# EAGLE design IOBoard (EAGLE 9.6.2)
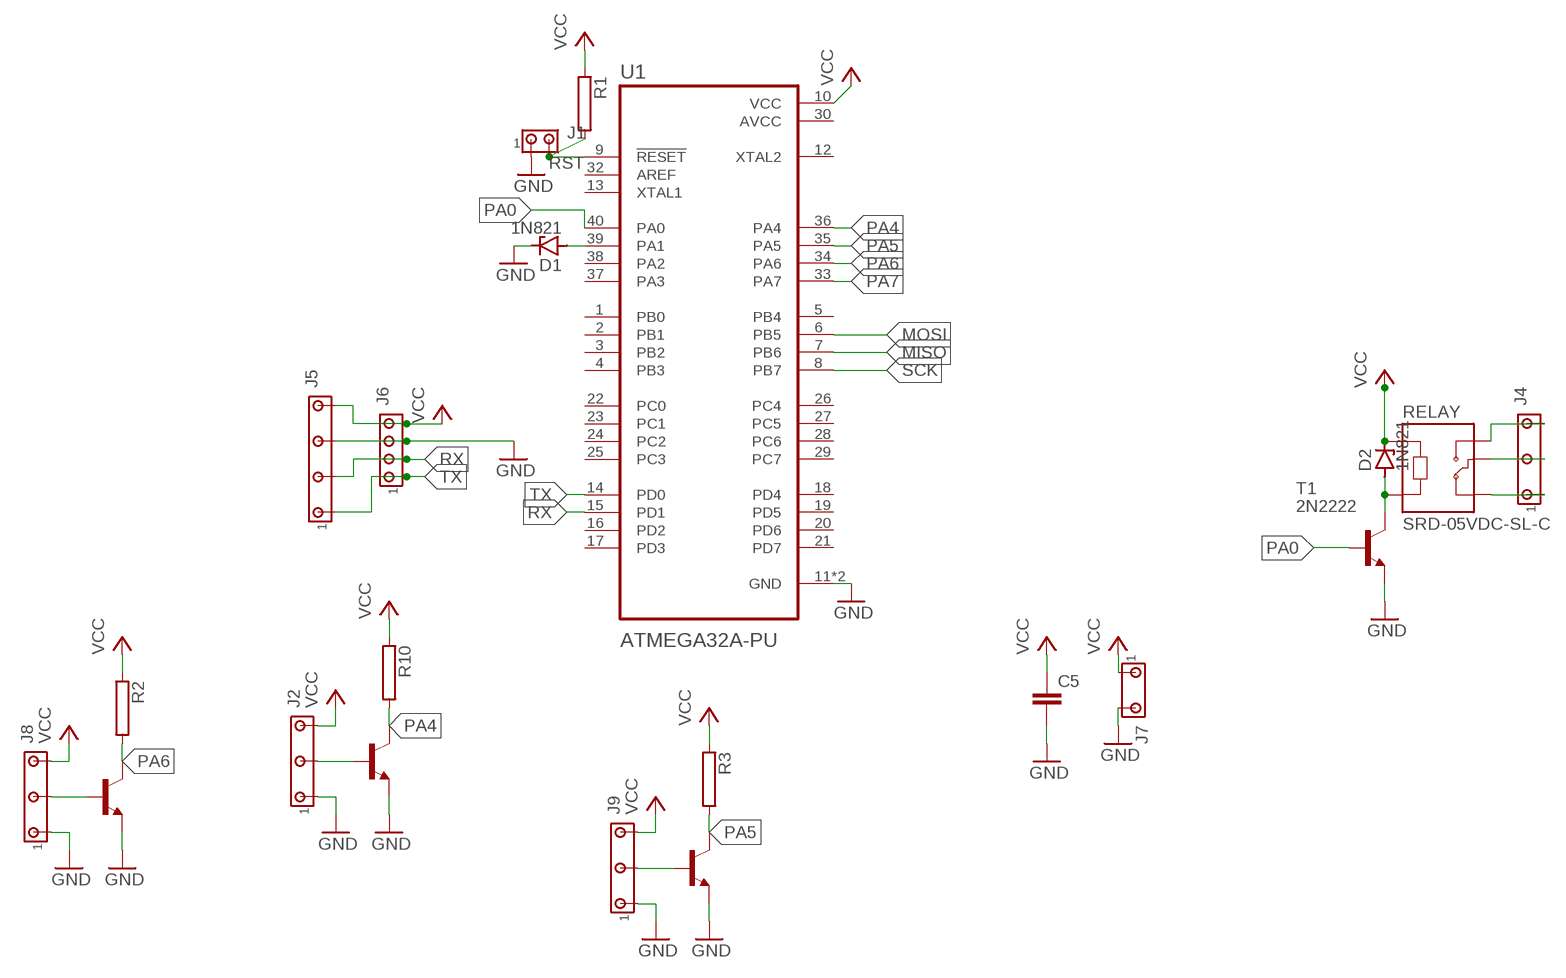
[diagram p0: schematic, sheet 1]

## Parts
C5  C-EU025-024X044  [C025-024X044]
D1  1N821  [DO35Z10]
D2  1N821  [DO35Z10]
J1  MTA02-100  [10X02MTA]
J2  MTA05-156_MYVSPACE1  [10X05MTA_MYV]
J4  MTA05-156_MYVSPACE1  [10X05MTA_MYV]
J5  MTA07-100_MYV  [10X07MTA_MYV]
J6  MTA04-100  [10X04MTA]
J7  MTA03-100_MYV  [10X03MTA_MYV]
J8  MTA05-156_MYVSPACE1  [10X05MTA_MYV]
J9  MTA05-156_MYVSPACE1  [10X05MTA_MYV]
R1  RHPS58  [HPS58]
R2  RHPS58  [HPS58]
R3  RHPS58  [HPS58]
R10  RHPS58  [HPS58]
RELAY  SRD-05VDC-SL-C  [RELAY_SRD-05VDC-SL-C]
T1  2N2222  [TO18]
T2  2N2222  [TO18]
T5  2N2222  [TO18]
T6  2N2222  [TO18]
U1  ATMEGA32A-PU  [DIP1540W47P254L5320H635Q40B]

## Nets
GND: C5.2 D1.C J1.1 J2.1 J5.5 J6.3 J7.3 J8.1 J9.1 T1.1(E) T2.1(E) T5.1(E) T6.1(E) U1.11(GND) U1.31(GND)
MISO: U1.7(PB6)
MOSI: U1.6(PB5)
N$1: J4.5 RELAY.NO
N$2: J4.3 RELAY.COM
N$3: J4.1 RELAY.NC
N$4: D2.A RELAY.A2 T1.3(C)
N$5: J8.3 T5.2(B)
N$6: J2.3 T2.2(B)
N$7: J9.3 T6.2(B)
PA0: T1.2(B) U1.40(PA0)
PA1: D1.A U1.39(PA1)
PA4: R10.2 T2.3(C) U1.36(PA4)
PA5: R3.2 T6.3(C) U1.35(PA5)
PA6: R2.2 T5.3(C) U1.34(PA6)
PA7: U1.33(PA7)
RST: J1.2 R1.2 U1.9(!RESET)
RX: J5.3 J6.2 U1.15(PD1)
SCK: U1.8(PB7)
TX: J5.1 J6.1 U1.14(PD0)
VCC: C5.1 D2.C J2.5 J5.7 J6.4 J7.1 J8.5 J9.5 R1.1 R2.1 R3.1 R10.1 RELAY.A1 U1.10(VCC)
Unconnected: U1.1(PB0) U1.2(PB1) U1.3(PB2) U1.4(PB3) U1.5(PB4) U1.12(XTAL2) U1.13(XTAL1) U1.16(PD2) U1.17(PD3) U1.18(PD4) U1.19(PD5) U1.20(PD6) U1.21(PD7) U1.22(PC0) U1.23(PC1) U1.24(PC2) U1.25(PC3) U1.26(PC4) U1.27(PC5) U1.28(PC6) U1.29(PC7) U1.32(AREF) U1.37(PA3) U1.38(PA2)

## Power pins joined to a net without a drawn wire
AVCC: U1.30(AVCC)

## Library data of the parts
C5 = rcl:C-EU: CAPACITOR, European symbol; SPICEPREFIX: C
D1 D2 = diode:1N821: Reference DIODE
J1 = con-amp:MTA02-100: AMP connector
J2 J4 J8 J9 = con-amp_edit:MTA05-156_MYV: AMP connector
J5 = con-amp_edit:MTA07-100_MYV: AMP connector
J6 = con-amp:MTA04-100: AMP connector
J7 = con-amp_edit:MTA03-100_MYV: AMP connector
R1-R3 R10 = resistor-power:R: Power Resitor; OC_FARNELL: unknown; OC_NEWARK: unknown
RELAY = SRD-05VDC-SL-C:SRD-05VDC-SL-C: 5V Trigger Relay Module For Arduino And Raspberry Pi 5V Trigger Relay Module For Arduino And Raspberry Pi; AVAILABILITY: Unavailable; DESCRIPTION: 5V Trigger Relay Module For Arduino And Raspberry Pi 5V Trigger Relay Module For Arduino And Raspberry Pi; MF: Songle Relay; MP: SRD-05VDC-SL-C; PACKAGE: None; PRICE: None
T1 T2 T5 T6 = transistor:2N2222: NPN TRANSISTOR
U1 = ATMEGA32A-PU:ATMEGA32A-PU; AVAILABILITY: Unavailable; DESCRIPTION: IC MCU 8BIT 32KB FLASH 40DIP; MF: Microchip Technology; MP: ATMEGA32A-PU; PACKAGE: None; PRICE: None

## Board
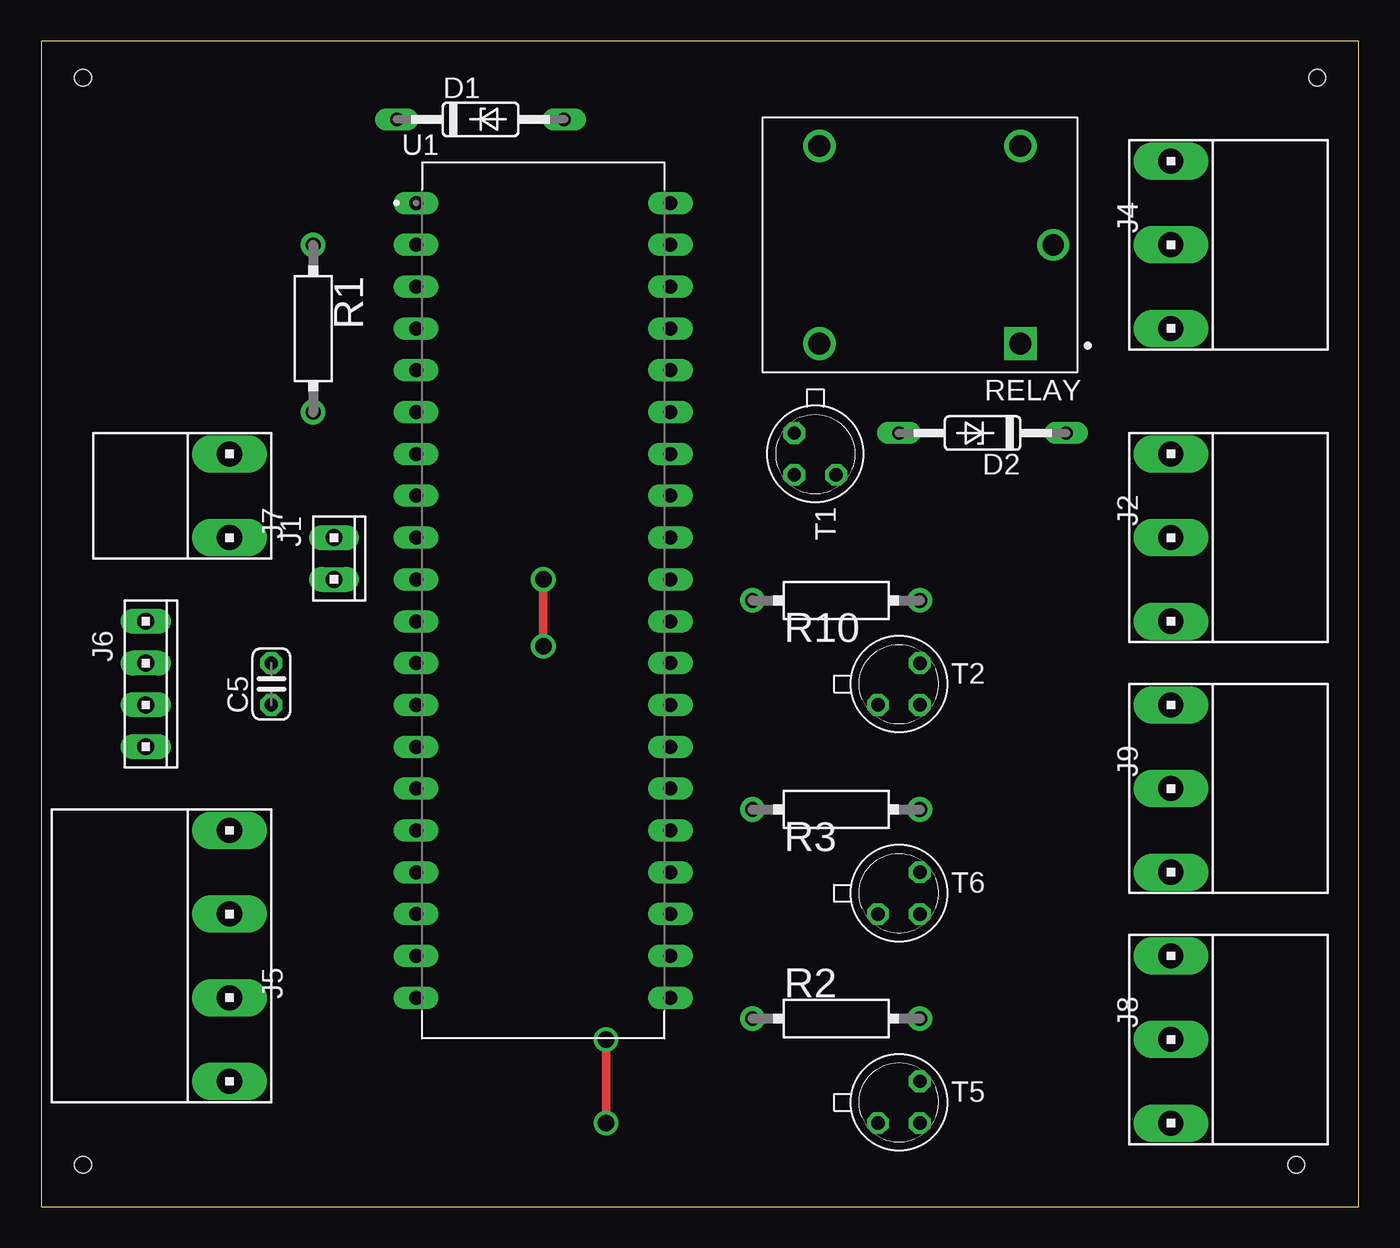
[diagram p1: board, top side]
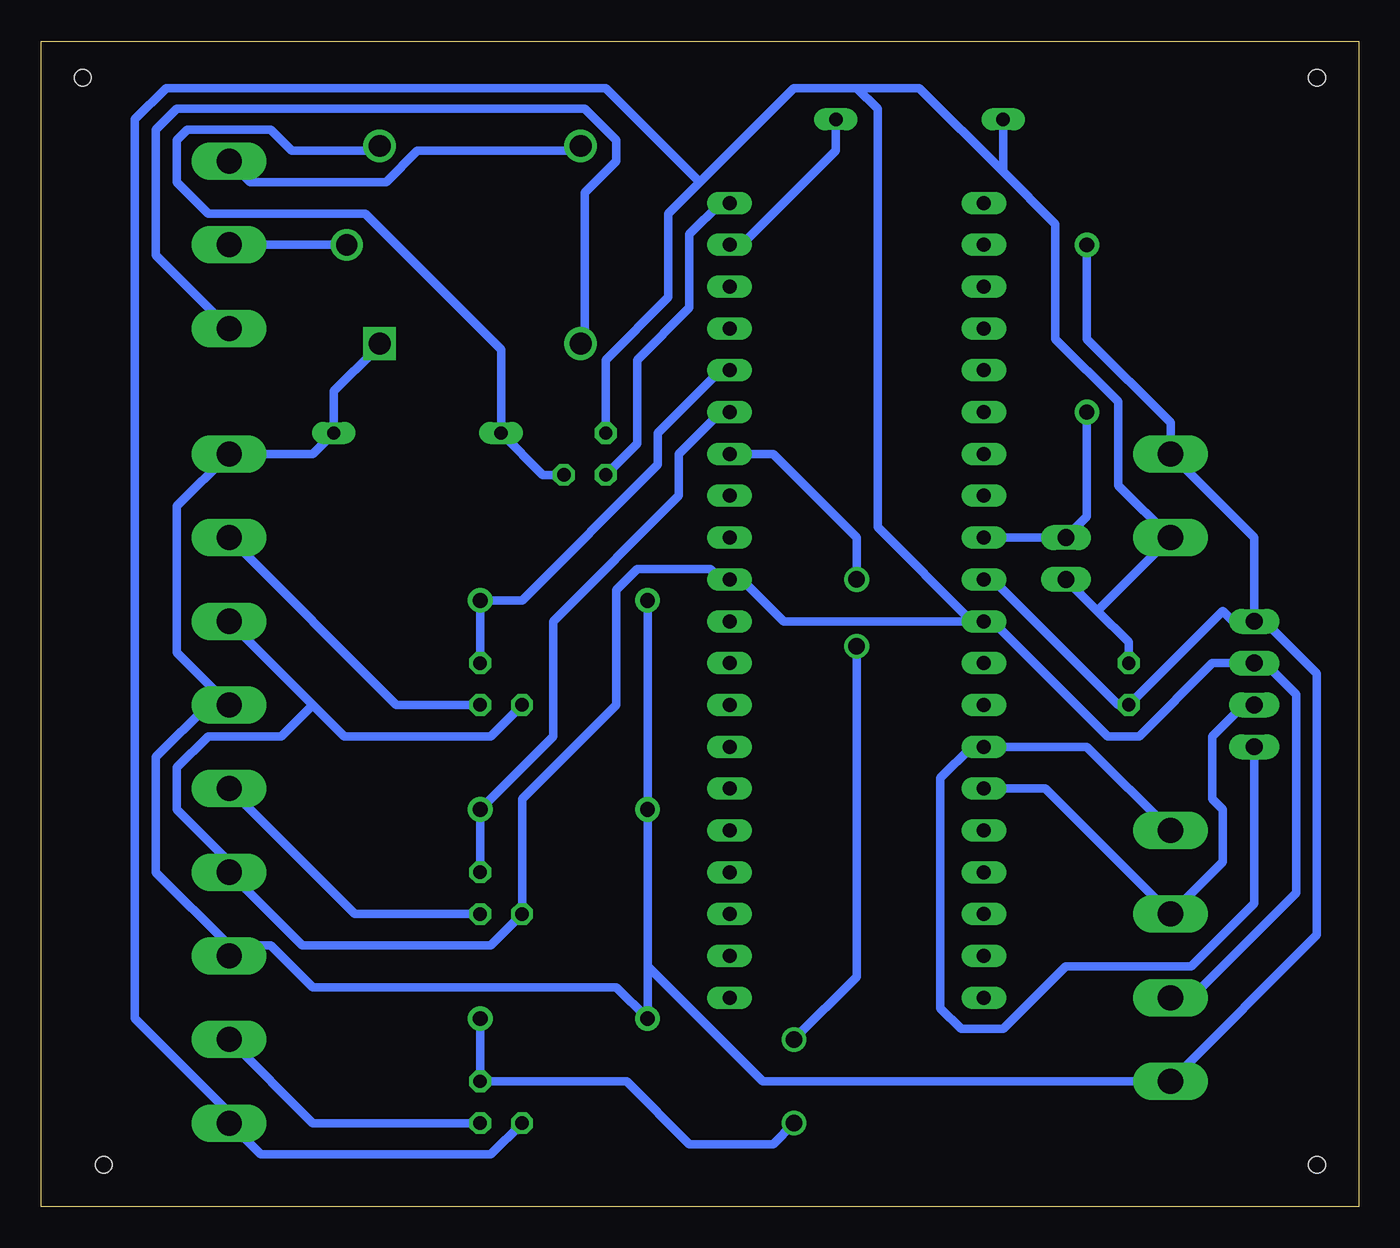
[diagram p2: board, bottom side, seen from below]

Size 79.99 x 70.79 mm. Coordinates in mm from the lower left corner, seen from the top.
Outline: 0,0 79.99,0 79.99,70.79 0,70.79 0,0
Copper layers (1*16): Top 0.035mm / dielectric 1.5mm / Bottom 0.035mm
Design rules "default *": minimum track width 20mil, minimum drill 0.35mm, track to track 20mil, track to pad 20mil, pad to pad 20mil, via to via 20mil, smd to smd 20mil, copper to edge 40mil, drill to drill 6mil, minimum pad ring 10mil, minimum via ring 8mil, stop-mask expansion 4mil, vias tented up to drill 0mil, thermal gap 10mil
Holes 1 mm at 2.54,68.58 77.47,68.58 2.54,2.54 76.2,2.54

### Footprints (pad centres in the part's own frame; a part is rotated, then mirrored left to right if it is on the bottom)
C025-024X044 = drill 0.813 octagon: 1 -1.27,0; 2 1.27,0
DO35Z10 = drill 0.813 long: A 5.08,0; C -5.08,0
10X02MTA = drill 1.016 long: 1 1.27,0; 2 -1.27,0
10X05MTA_MYV = drill 1.524 long: 1 5.08,0; 3 0,0; 5 -5.08,0
10X07MTA_MYV = drill 1.524 long: 1 7.62,0; 3 2.54,0; 5 -2.54,0; 7 -7.62,0
10X04MTA = drill 1.016 long: 1 3.81,0; 2 1.27,0; 3 -1.27,0; 4 -3.81,0
10X03MTA_MYV = drill 1.524 long: 1 2.54,0; 3 -2.54,0
HPS58 = drill 0.9 pad 1.5: 1 -5.08,0; 2 5.08,0
RELAY_SRD-05VDC-SL-C = drill 1.32 square: A1 -6.1,6 | drill 1.32: A2 -6.1,-6; NC 6.1,6; NO 6.1,-6 | drill 1.29: COM -8.1,0
TO18 = drill 0.813 octagon: 1 -1.27,-1.27; 2 1.27,-1.27; 3 1.27,1.27
DIP1540W47P254L5320H635Q40B = drill 0.85 pad 1.28 long: 1 -7.718,24.13; 2 -7.718,21.59; 3 -7.718,19.05; 4 -7.718,16.51; 5 -7.718,13.97; 6 -7.718,11.43; 7 -7.718,8.89; 8 -7.718,6.35; 9 -7.718,3.81; 10 -7.718,1.27; 11 -7.718,-1.27; 12 -7.718,-3.81; 13 -7.718,-6.35; 14 -7.718,-8.89; 15 -7.718,-11.43; 16 -7.718,-13.97; 17 -7.718,-16.51; 18 -7.718,-19.05; 19 -7.718,-21.59; 20 -7.718,-24.13; 21 7.718,-24.13; 22 7.718,-21.59; 23 7.718,-19.05; 24 7.718,-16.51; 25 7.718,-13.97; 26 7.718,-11.43; 27 7.718,-8.89; 28 7.718,-6.35; 29 7.718,-3.81; 30 7.718,-1.27; 31 7.718,1.27; 32 7.718,3.81; 33 7.718,6.35; 34 7.718,8.89; 35 7.718,11.43; 36 7.718,13.97; 37 7.718,16.51; 38 7.718,19.05; 39 7.718,21.59; 40 7.718,24.13

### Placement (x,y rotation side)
C5  13.97,31.75 90 top
D1  26.67,66.04 0 top
D2  57.15,46.99 180 top
J1  17.78,39.37 270 top
J2  68.58,40.64 270 top
J4  68.58,58.42 270 top
J5  11.43,15.24 90 top
J6  6.35,31.75 270 top
J7  11.43,43.18 90 top
J8  68.58,10.16 270 top
J9  68.58,25.4 270 top
R1  16.51,53.34 270 top
R2  48.26,11.43 0 top
R3  48.26,24.13 0 top
R10  48.26,36.83 0 top
RELAY  53.34,58.42 180 top
T1  46.99,45.72 270 top
T2  52.07,31.75 0 top
T5  52.07,6.35 0 top
T6  52.07,19.05 0 top
U1  30.48,36.83 0 top

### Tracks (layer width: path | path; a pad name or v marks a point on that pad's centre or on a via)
GND
  Bottom 0.508: T2.1 52.7,28.57 61.59,28.57 63.5,30.48 | J2.1 63.5,30.48 | 63.5,30.48 65.41,28.57 69.85,28.57 71.75,26.67 71.75,24.13 68.58,20.95 J9.1 64.14,15.88 52.7,15.88 T6.1 50.8,24.77 45.09,30.48 45.09,37.47 43.81,38.73 39.37,38.73 38.73,38.1 U1.31 37.47,38.1 34.92,35.56 23.5,35.56 | J5.5 10.16,12.7 3.81,19.05 3.81,31.11 5.71,33.02 J6.3 8.89,33.02 13.34,28.57 15.24,28.57 22.23,35.56 U1.11 23.5,35.56 | T5.1 52.7,3.17 66.67,3.17 J8.1 68.58,5.71 74.3,11.43 74.3,66.04 72.39,67.94 45.72,67.94 40.01,62.23 | C5.2 13.97,34.29 15.88,36.2 | J1.1 15.88,36.2 | 21.59,62.87 D1.C | 21.59,62.87 18.41,59.69 18.41,52.7 14.61,48.9 14.61,43.81 J7.3 15.88,36.2 | T1.1 45.72,51.44 41.91,55.24 41.91,60.33 40.01,62.23 | 40.01,62.23 34.29,67.94 30.48,67.94 | 30.48,67.94 26.67,67.94 21.59,62.87 | 23.5,35.56 29.21,41.27 29.21,66.67 30.48,67.94
N$1
  Bottom 0.508: J4.5 67.31,62.23 59.05,62.23 57.15,64.14 47.62,64.14 RELAY.NO
N$2
  Bottom 0.508: J4.3 RELAY.COM
N$3
  Bottom 0.508: J4.1 73.03,57.78 73.03,65.41 71.75,66.67 46.99,66.67 45.09,64.77 45.09,63.5 46.99,61.59 46.99,52.7 RELAY.NC
N$4
  Bottom 0.508: T1.3 49.53,44.45 D2.A 52.07,52.07 60.33,60.33 69.85,60.33 71.75,62.23 71.75,64.77 71.12,65.41 66.04,65.41 64.77,64.14 59.69,64.14 RELAY.A2
N$5
  Bottom 0.508: T5.2 63.5,5.08 J8.3
N$6
  Bottom 0.508: T2.2 58.42,30.48 J2.3
N$7
  Bottom 0.508: T6.2 60.96,17.78 J9.3
PA0
  Bottom 0.508: T1.2 43.81,46.35 43.81,51.44 40.64,54.61 40.64,59.05 38.73,60.96 U1.40
PA1
  Bottom 0.508: D1.A 31.75,64.14 37.47,58.42 U1.39
PA4
  Bottom 0.508: T2.3 R10.2 50.8,36.83 42.55,45.09 42.55,46.99 38.73,50.8 U1.36
PA5
  Bottom 0.508: T6.3 R3.2 48.9,28.57 48.9,35.56 41.27,43.18 41.27,45.72 38.73,48.26 U1.35
PA6  (via drill 1)
  Top 0.508: v34.29,5.08 v34.29,10.16 | v30.48,38.1 v30.48,34.05
  Bottom 0.508: R2.2 T5.3 44.45,7.62 40.64,3.81 35.56,3.81 v34.29,5.08 | v34.29,10.16 30.48,13.97 v30.48,34.05 | v30.48,38.1 30.48,40.64 35.56,45.72 U1.34
RST
  Bottom 0.508: U1.9 J1.2 16.51,41.91 R1.2
RX
  Bottom 0.508: U1.15 19.05,25.4 J5.3 8.26,20.95 8.26,24.13 8.89,24.77 8.89,28.57 6.99,30.48 J6.2
TX
  Bottom 0.508: J5.1 16.51,27.94 U1.14 23.5,27.94 25.4,26.04 25.4,12.06 24.13,10.79 21.59,10.79 17.78,14.61 10.16,14.61 6.35,18.41 J6.1
VCC
  Bottom 0.508: RELAY.A1 59.69,52.07 62.23,49.53 D2.C 63.5,45.72 J2.5 71.75,42.55 71.75,33.66 J9.5 69.85,30.48 73.03,27.3 73.03,20.32 68.58,15.88 | U1.10 22.23,38.1 14.61,30.48 C5.1 8.26,36.2 7.62,35.56 J6.4 6.35,36.2 | R1.1 16.51,52.7 11.43,47.62 J7.1 6.35,40.64 6.35,36.2 | 43.18,14.61 R3.1 R10.1 | 43.18,14.61 R2.1 45.09,13.34 63.5,13.34 66.04,15.88 68.58,15.88 | 43.18,14.61 36.2,7.62 J5.7 2.54,16.51 2.54,32.38 6.35,36.2 | 68.58,15.88 J8.5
